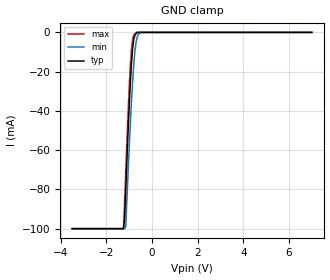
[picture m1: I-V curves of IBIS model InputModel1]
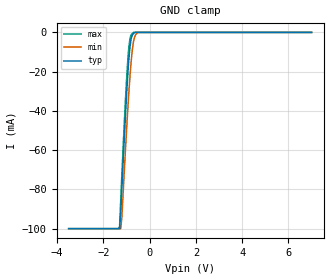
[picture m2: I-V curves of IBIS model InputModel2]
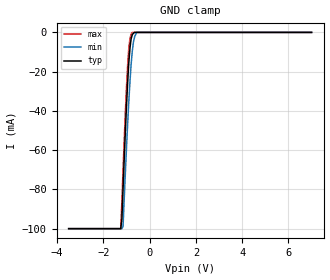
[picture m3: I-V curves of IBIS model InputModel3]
[IBIS Ver]   2.1
[File name]   pa008sal.ibs  | pa= PSOP, f0008sa-l= abbr chip name, 3=3.3V Vcc
[File Rev]   2.00
[Date]   3-April-96
[Source]   File generated from lab measurements at Intel Corporation
[Notes]   Rev 2.00 All data was replaced by actual measurements
   performed in a lab.
[Disclaimer] INTEL DEVELOPER'S SOFTWARE LICENSE AGREEMENT
| BY USING THIS SOFTWARE, YOU ARE AGREEING TO BE BOUND
| BY THE TERMS OF THIS AGREEMENT.  DO NOT USE THE SOFTWARE
| UNTIL YOU HAVE CAREFULLY READ AND AGREED TO THE FOLLOWING
| TERMS AND CONDITIONS.  IF YOU DO NOT AGREE TO THE TERMS
| OF THIS AGREEMENT, PROMPTLY RETURN THE SOFTWARE PACKAGE
| AND ANY ACCOMPANYING ITEMS.
| IF YOU USE THIS SOFTWARE, YOU WILL BE BOUND BY THE TERMS
| OF THIS AGREEMENT
| LICENSE: Intel Corporation ("Intel") grants you the non-exclusive right
| to use the enclosed software program ("Software").  You will not use,
| copy, modify, rent, sell or transfer the Software or any portion
| thereof, except as provided in this Agreement.
| System OEM Developers may:
| 1.   Copy the Software for support, backup or archival purposes;
| 2.   Install, use, or distribute Intel owned Software in object code
|   only;
| 3.   Modify and/or use Software source code that Intel directly makes
|   available to you as an OEM Developer;
| 4.   Install, use, modify, distribute, and/or make or have made
|   derivatives ("Derivatives") of Intel owned Software under the
|   terms and conditions in this Agreement, ONLY if you are a System
|   OEM Developer and NOT an end-user.
| RESTRICTIONS:
| YOU WILL NOT:
| 1.   Copy the Software, in whole or in part, except as provided for
|   in this Agreement;
| 2.   Decompile or reverse engineer any Software provided in object
|   code format;
| 3.   Distribute any Software or Derivative code to any end-users,
|   unless approved by Intel in a prior writing.
| TRANSFER: You may transfer the Software to another OEM
| Developer if the receiving party agrees to the terms of this
| Agreement at the sole risk of any receiving party.
| OWNERSHIP AND COPYRIGHT OF SOFTWARE:
| Title to the Software and all copies thereof remain with Intel
| or its vendors.  The Software is copyrighted and is protected by
| United States and international copyright laws.  You will not
| remove the copyright notice from the Software.  You agree to
| prevent any unauthorized copying of the Software.
| DERIVATIVE WORK: OEM Developers that make or have made
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[Copyright]   Copyright 1996, Intel Corporation, All Rights Reserved
[Component]   PA28F008SA-L   | 44-lead PSOP package, 28F008SA-L
[Manufacturer]  Intel   | Flash File (tm)
|   | operating in 3.3 V Vcc range
[Package]
|The following values apply for the leadframe.
|Variable   typ   min   max
R_pkg   145.5m   144.0m   147.0m
L_pkg   5.25nH   2.00nH   8.50nH
C_pkg   1.09pF   0.68pF   1.50pF
|*****************************Pin Definitions**********************************
[Pin]   signal_name   model_name   R_pin   L_pin   C_pin
  1   VPP   POWER
  2   RP#   InputModel4
  3   A11   InputModel2
  4   A10   InputModel2
  5   A09   InputModel2
  6   A08   InputModel2
  7   A07   InputModel2
  8   A06   InputModel2
  9   A05   InputModel2
 10   A04   InputModel2
 11   NC   InputModel5
 12   NC   InputModel5
 13   A03   InputModel1
 14   A02   InputModel1
 15   A01   InputModel1
 16   A00   InputModel1
 17   DQ0   InputOutput
 18   DQ1   InputOutput
 19   DQ2   InputOutput
 20   DQ3   InputOutput
 21   GND   GND
 22   GND   GND
 23   VCC   POWER
 24   DQ4   InputOutput
 25   DQ5   InputOutput
 26   DQ6   InputOutput
 27   DQ7   InputOutput
 28   RY/BY#   RYBYOutput
 29   OE#   InputModel3
 30   WE#   InputModel3
 31   NC   InputModel5
 32   NC   InputModel5
 33   NC   InputModel5
 34   NC   InputModel5
 35   A19   InputModel2
 36   A18   InputModel2
 37   A17   InputModel2
 38   A16   InputModel2
 39   A15   InputModel2
 40   A14   InputModel2
 41   A13   InputModel2
 42   A12   InputModel2
 43   CE#   InputModel3
 44   VCC   POWER
|**********************Input Model 5***************************************
[Model]   InputModel5
Model_type   Input
|   For NC pins
Vinl = 0.8V
Vinh = 2.0V
| Variable   typ   min   max
C_comp   5.61p   NA   7.6p
[Voltage Range]   3.3V   3.0V   3.6V
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| Models and submodels in the file (7): InputModel1 (Input), InputModel2 (Input), InputModel3 (Input), InputModel4 (Input), InputModel5 (Input), InputOutput (I/O), RYBYOutput (Output)
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|**************************Input Model 1***************************************
[Model]   InputModel1
Model_type   Input
|   For A[3:0]
Vinl = 0.8V
Vinh = 2.0V
| Variable   typ   min   max
C_comp   5.61p   NA   7.6p
[Voltage Range]   3.3V   3.0V   3.6V
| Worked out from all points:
|   GND clamp passes 1 mA (typ) near -0.72 V on its own axis
[GND_clamp]
|Voltage I(typ)   I(min)   I(max)
-3.5V     -100mA     -100mA     -100mA
-1.25V    -100mA     -100mA     -100mA
-1.2V     -95.07mA   -100mA     -86.07mA
-1.15V    -79.86mA   -99mA      -70.4mA
-1.05V    -50.95mA   -71.8mA    -41.05mA
-950mV    -25.72mA   -46.61mA   -16.75mA
-900mV    -15.57mA   -35.21mA   -8.231mA
-850mV    -8.181mA   -25.25mA   -3.35mA
-800mV    -3.515mA   -16.43mA   -1.299mA
-700mV    -671.7uA   -5.073mA   0A
-500mV    0A         0A         0A
7V        0A         0A         0A
[POWER_clamp]
| Input buffer circuits of this product do not intrinsically
| require a [POWER_clamp] definition.  This zero current
| [POWER_clamp] is provided for compatibility with some ibis
| parsers.
|Voltage  I(typ)   I(min)   I(max)
-3.3V     0A         0A         0A
0V        0A         0A         0A
3.3V      0A         0A         0A
6.6V      0A         0A         0A
|**********************Input Model 2************************************
[Model]   InputModel2
Model_type   Input
|   For A[19:4]
Vinl = 0.8V
Vinh = 2.0V
| Variable   typ   min   max
C_comp   5.61p   NA   7.6p
[Voltage Range]   3.3V   3.0V   3.6V
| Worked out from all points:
|   GND clamp passes 1 mA (typ) near -0.73 V on its own axis
[GND_clamp]
|Voltage I(typ)   I(min)   I(max)
-3.5V     -100mA     -100mA     -100mA
-1.3V     -100mA     -100mA     -99.05mA
-1.25V    -91.91mA   -100mA     -85.56mA
-1.2V     -79.19mA   -94.07mA   -72.29mA
-1.05V    -43.33mA   -60.73mA   -35.37mA
-950mV    -22.48mA   -40.12mA   -14.99mA
-900mV    -13.9mA    -30.69mA   -7.576mA
-850mV    -7.472mA   -22.37mA   -3.135mA
-800mV    -3.262mA   -14.88mA   -1.175mA
-700mV    -582uA     -4.802mA   0A
-500mV    0A         0A         0A
7V        0A         0A         0A
[POWER_clamp]
| Input buffer circuits of this product do not intrinsically
| require a [POWER_clamp] definition.  This zero current
| [POWER_clamp] is provided for compatibility with some ibis
| parsers.
|Voltage  I(typ)   I(min)   I(max)
-3.3V     0A         0A         0A
0V        0A         0A         0A
3.3V      0A         0A         0A
6.6V      0A         0A         0A
|*********************Input Model 3**************************************
[Model]   InputModel3
Model_type   Input
|   For WE#, OE# & CE#
Vinl = 0.8V
Vinh = 2.0V
| Variable   typ   min   max
C_comp   5.61p   NA   7.6p
[Voltage Range]   3.3V   3.0V   3.6V
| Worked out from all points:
|   GND clamp passes 1 mA (typ) near -0.74 V on its own axis
[GND_clamp]
|Voltage I(typ)   I(min)   I(max)
-3.5V     -100mA     -100mA     -100mA
-1.25V    -100mA     -100mA     -100mA
-1.2V     -95.1mA    -100mA     -86.12mA
-1.15V    -79.72mA   -98.88mA   -70.26mA
-1.05V    -50.65mA   -71.61mA   -40.78mA
-950mV    -25.39mA   -46.36mA   -16.47mA
-900mV    -15.22mA   -34.94mA   -7.948mA
-850mV    -7.856mA   -24.98mA   -3.051mA
-750mV    -1.172mA   -9.488mA   0A
-650mV    0A         -2.268mA   0A
-550mV    0A         0A         0A
7V        0A         0A         0A
[POWER_clamp]
| Input buffer circuits of this product do not intrinsically
| require a [POWER_clamp] definition.  This zero current
| [POWER_clamp] is provided for compatibility with some ibis
| parsers.
|Voltage  I(typ)   I(min)   I(max)
-3.3V     0A         0A         0A
0V        0A         0A         0A
3.3V      0A         0A         0A
6.6V      0A         0A         0A
